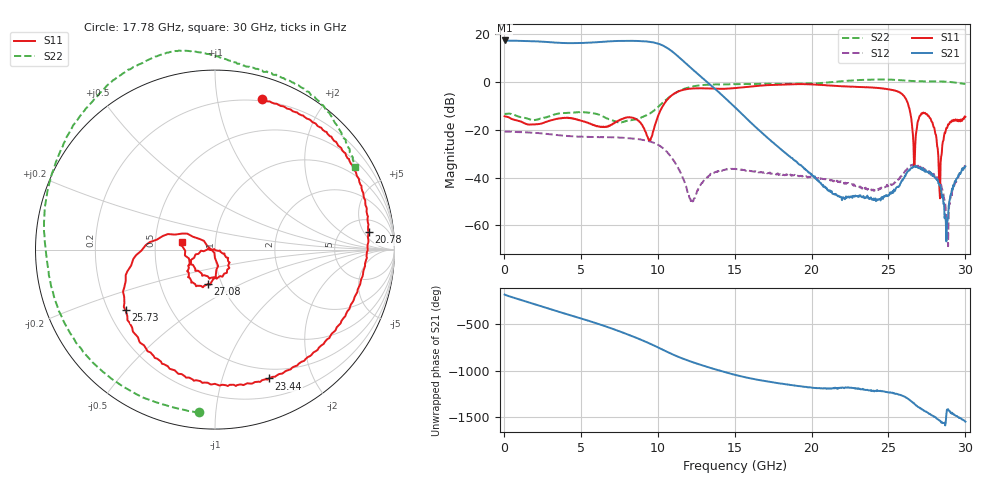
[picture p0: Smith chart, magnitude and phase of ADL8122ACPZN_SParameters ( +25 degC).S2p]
! "Analog Devices, Inc."
! Device:	ADL8122ACPZN
! Description:	"10 kHz to 10 GHz, Wideband, Low Noise Amplifier"
! Conditions:	Vdd = 5.0 V
!		IDQ = 95 mA
!		Pin = -25 dBm
!		Operating Temperature = +25 C (at package bottom)
! Product validation unit SN1 soldered down to Evaluation Board as shown on ADL8122-EVALZ User Guide. Board loss de-embedded from S21 magnitude.  All other RF measurements reference to RF coaxial connector.
! Frequency (GHz)	S11_Mag (dB)	S11_Phase (deg)	S21_Mag (dB)	S21_Phase (deg)	S12_Mag (dB)	S12_Phase (deg)	S22_Mag (dB)	S22_Phase (deg)
#  GHZ  S  DB  R 50
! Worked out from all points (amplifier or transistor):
!   800 points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, 37.51 MHz to 30 GHz, reference 50 ohm
!   highest |S21| = 17.4 dB at 37.51 MHz (marker M1)
!   |S21| within 3 dB of that: start of sweep to 10.58 GHz
!   unconditionally stable (mu >= 1): start of sweep to 21.33 GHz; 29 GHz to end of sweep
!   at 5.025 GHz: K = 1.24, MAG = 16.6 dB, |S12| = -22.9 dB
!   at 15.04 GHz: K = 8.97, MAG = 0.3 dB, |S12| = -36.3 dB
!   at 30 GHz: K = 287.52, MAG = -27.7 dB, |S12| = -35.1 dB
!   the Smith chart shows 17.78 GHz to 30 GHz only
!   S11 on the Smith chart (normalised r, x): 17.78 GHz: 0.19, +1.35; 20.78 GHz: 9, +6; 23.44 GHz: 0.39, -1.43; 25.73 GHz: 0.27, -0.29; 27.08 GHz: 0.86, -0.34; 30 GHz: 0.69, +0.06
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0.03750899  -14.33 -172.8  17.36 -178.9  -20.71 1.8  -13.16 170.6
1.087509  -16.55 158.2  17.18 123.4  -20.99 -48.8  -14.68 104.3
1.912508  -17.74 157.6  17.04 80.3  -21.22 -86.1  -15.99 37.2
3.412508  -15.47 130.6  16.44 3.5  -22.18 -154.1  -13.38 -71.4
5.062508  -16.34 43.0  16.32 -78.4  -22.89 131.3  -12.60 -125.3
5.962507  -18.28 0.4  16.59 -125.4  -23.03 88.1  -13.30 -156.9
6.900007  -18.24 -14.9  16.99 -177.9  -23.12 40.9  -15.75 145.7
8.287506  -14.85 -60.1  17.21 96.6  -23.60 -33.6  -15.90 28.0
9.300006  -22.58 -146.7  16.92 27.5  -24.60 -93.4  -13.80 -36.7
10.05001  -13.64 65.3  15.96 -30.0  -26.41 -143.6  -10.19 -93.8
10.61251  -7.42 22.3  14.21 -75.2  -29.38 175.6  -7.05 -142.8
11.43751  -3.72 -27.0  10.00 -135.7  -37.49 115.4  -3.59 154.4
12.71251  -2.66 -88.0  2.73 149.6  -43.59 -83.5  -1.43 84.3
15.0375  -2.55 162.8  -10.69 37.1  -36.32 158.4  -0.91 -18.2
17.775  -1.14 72.5  -26.94 -49.9  -38.30 80.0  -0.81 -95.5
20.025  -1.04 24.0  -38.99 -99.6  -39.71 23.8  -0.60 -165.1
20.775  -1.29 6.5  -43.89 -104.7  -40.56 3.1  -0.34 171.9
23.4375  -2.18 -67.3  -48.63 -120.9  -44.45 -69.5  0.89 117.2
25.0125  -3.11 -114.1  -47.50 -152.0  -43.09 -111.7  1.01 99.2
25.725  -4.41 -145.9  -43.33 -175.5  -40.03 -145.7  0.76 92.4
27.075  -14.06 -102.2  -36.32 35.6  -35.42 49.8  0.30 78.0
30  -14.59 166.7  -35.29 -104.6  -35.07 -99.7  -0.87 30.4
